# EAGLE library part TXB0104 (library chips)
4-BIT BIDIRECTIONAL VOLTAGE-LEVEL TRANSLATOR
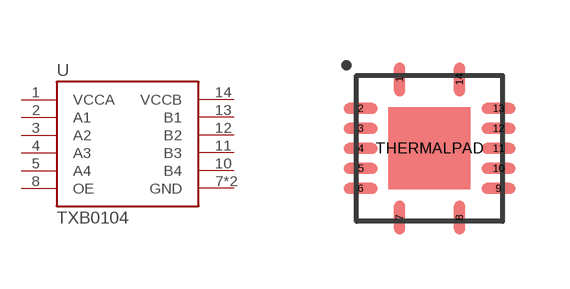
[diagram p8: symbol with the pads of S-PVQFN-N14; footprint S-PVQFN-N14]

Designator prefix U

## TXB0104RGY (DIGIKEY: 296-21930-1-ND)  [S-PVQFN-N14]
1  VCCA
2  A1
3  A2
4  A3
5  A4
7  GND
8  OE
10  B4
11  B3
12  B2
13  B1
14  VCCB
THERMALPAD  GND

## Footprint S-PVQFN-N14 (pad centres in mm)
smd 0.28 x 0.85: 1 -0.75,1.725; 7 -0.75,-1.725; 8 0.75,-1.725; 14 0.75,1.725
smd 0.85 x 0.28: 2 -1.725,1; 3 -1.725,0.5; 4 -1.725,0; 5 -1.725,-0.5; 6 -1.725,-1; 9 1.725,-1; 10 1.725,-0.5; 11 1.725,0; 12 1.725,0.5; 13 1.725,1
smd 2.05 x 2.05: THERMALPAD 0,0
